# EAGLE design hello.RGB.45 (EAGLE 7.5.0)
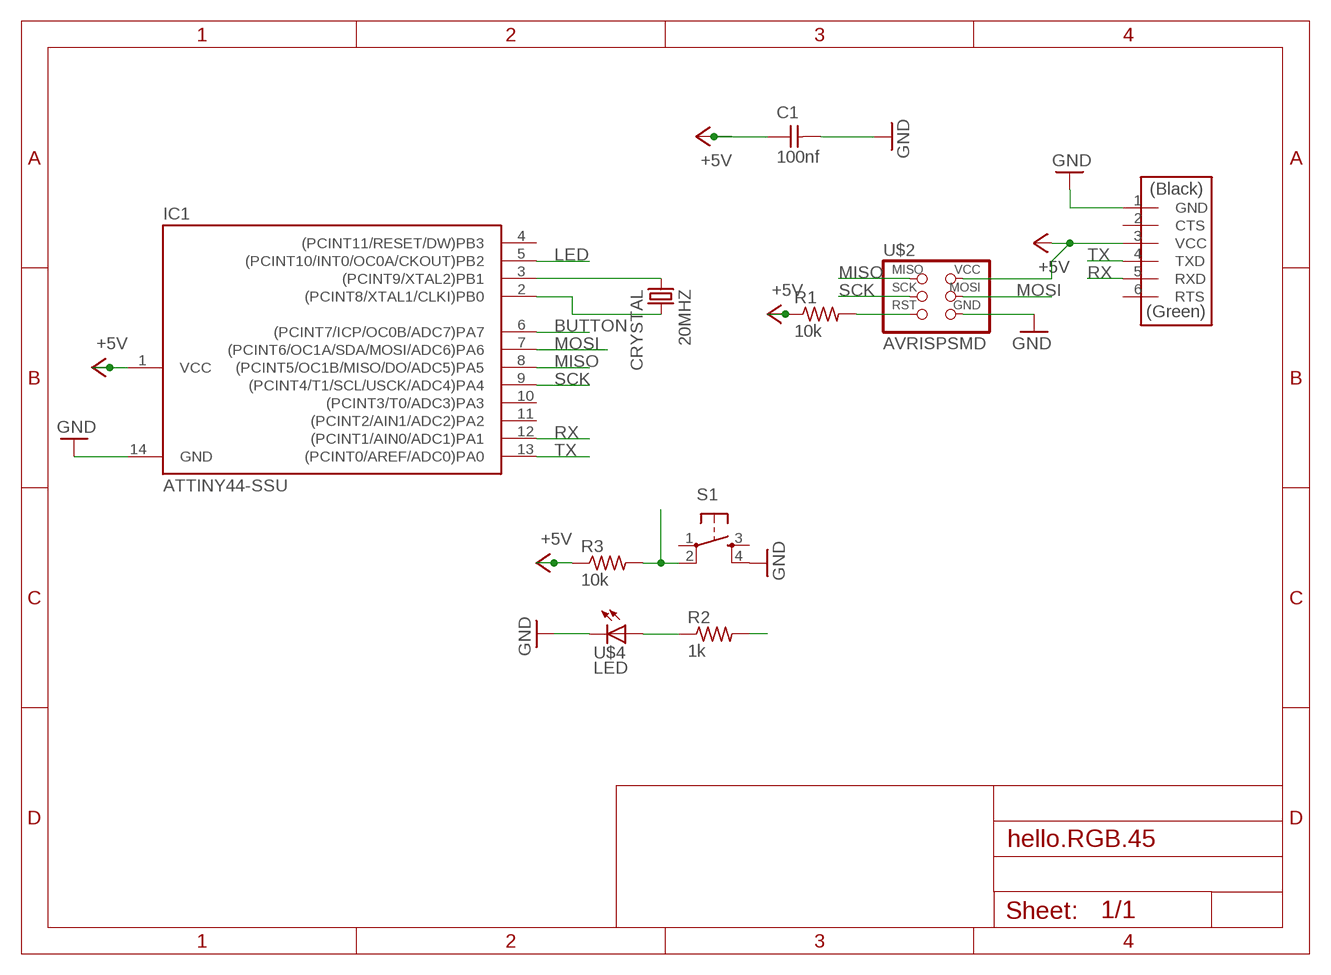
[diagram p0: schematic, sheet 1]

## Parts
20MHZ  CRYSTAL  [2-SMD-5X3MM]
C1  100nf  CAP-UNPOLARIZEDFAB  [C1206FAB]
IC1  ATTINY44-SSU  [SOIC14]
R1  10k  RES-US1206  [R1206]
R2  1k  RES-US1206  [R1206]
R3  10k  RES-US1206  [R1206]
S1  6MM_SWITCH6MM_SWITCH  [6MM_SWITCH]
U$1  FTDI-SMD-HEADER  [1X06SMD]
U$2  AVRISPSMD  [2X03SMD]
U$4  LED  [LED1206]

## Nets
+5V: C1.1 IC1.1(VCC) R1.1 R3.1 U$1.3(VCC) U$2.2(VCC)
BUTTON: IC1.6((PCINT7/ICP/OC0B/ADC7)PA7) R3.2 S1.2(P1)
GND: C1.2 IC1.14(GND) S1.4(S1) U$1.1(GND) U$2.6(GND) U$4.2(C)
LED: IC1.5((PCINT10/INT0/OC0A/CKOUT)PB2) R2.2
MISO: IC1.8((PCINT5/OC1B/MISO/DO/ADC5)PA5) U$2.1(MISO)
MOSI: IC1.7((PCINT6/OC1A/SDA/MOSI/ADC6)PA6) U$2.4(MOSI)
N$1: 20MHZ.P$2 IC1.2((PCINT8/XTAL1/CLKI)PB0)
N$2: 20MHZ.P$1 IC1.3((PCINT9/XTAL2)PB1)
N$11: R1.2 U$2.5(RST)
N$14: R2.1 U$4.1(A)
RX: IC1.12((PCINT1/AIN0/ADC1)PA1) U$1.5(RXD)
SCK: IC1.9((PCINT4/T1/SCL/USCK/ADC4)PA4) U$2.3(SCK)
TX: IC1.13((PCINT0/AREF/ADC0)PA0) U$1.4(TXD)
Unconnected: IC1.4((PCINT11/RESET/DW)PB3) IC1.10((PCINT3/T0/ADC3)PA3) IC1.11((PCINT2/AIN1/ADC2)PA2) S1.1(P) S1.3(S) U$1.2(CTS) U$1.6(RTS)

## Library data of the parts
20MHZ = fab:CRYSTAL
C1 = fab:CAP-UNPOLARIZED
IC1 = fab:ATTINY44
R1-R3 = fab:RES-US: Resistor (US Symbol)
S1 = fab:6MM_SWITCH: OMRON SWITCH
U$1 = fab:FTDI-SMD-HEADER
U$2 = fab:AVRISP
U$4 = fab:LED: LED

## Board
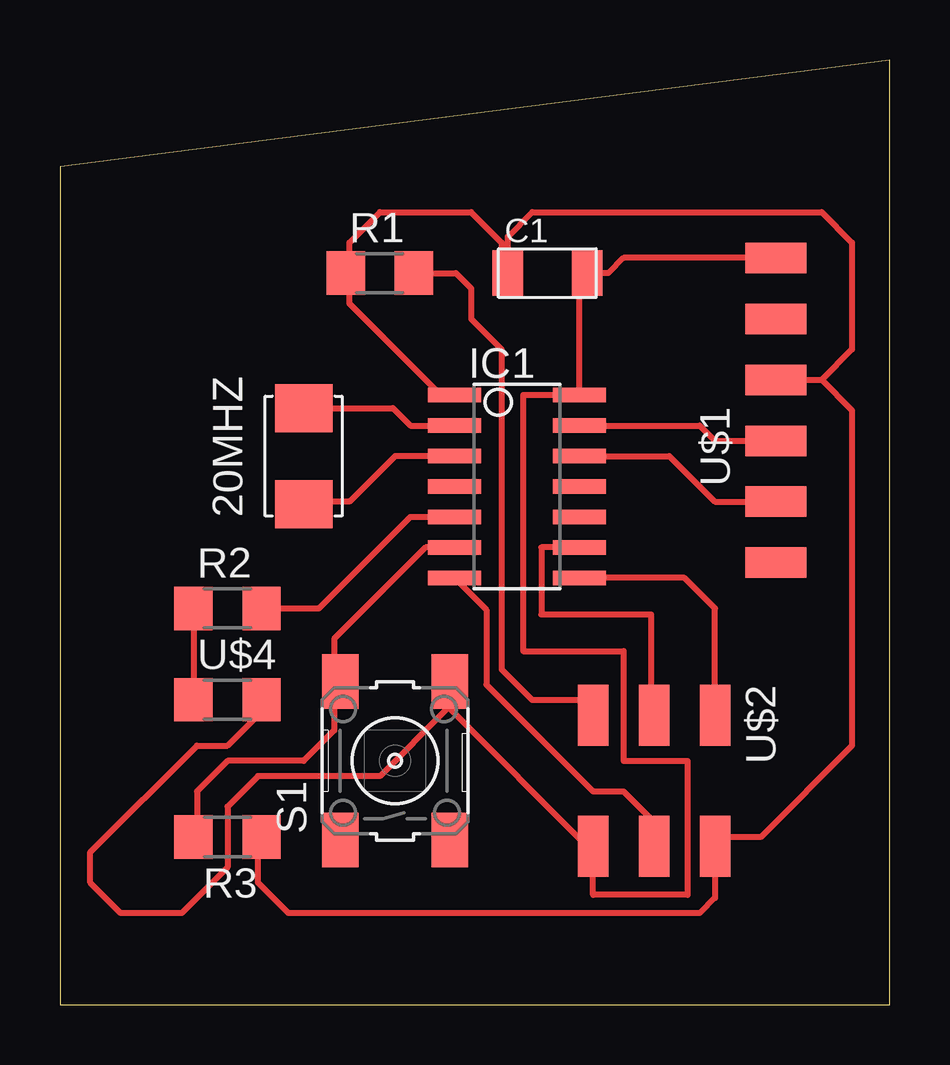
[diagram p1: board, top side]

Size 34.59 x 39.36 mm. Coordinates in mm from the lower left corner, seen from the top.
Outline: 0,0 34.59,0 34.59,39.36 0,34.92 0,0
Copper layers (1*16): Top 0.035mm / dielectric 1.5mm / Bottom 0.035mm
Design rules "default": minimum track width 10mil, minimum drill 24mil, track to track 8mil, track to pad 8mil, pad to pad 8mil, via to via 8mil, smd to smd 8mil, copper to edge 40mil, drill to drill 8mil, minimum pad ring 10mil, minimum via ring 8mil, stop-mask expansion 4mil, vias tented up to drill 0mil, thermal gap 10mil

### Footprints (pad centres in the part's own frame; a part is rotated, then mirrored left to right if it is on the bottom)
2-SMD-5X3MM = smd 2 x 2.4: P$1 -2,0; P$2 2,0
C1206FAB = smd 1.27 x 1.905: 1 -1.651,0; 2 1.651,0
SOIC14 = smd 0.61 x 2.21: 1 -3.81,-2.603; 2 -2.54,-2.603; 3 -1.27,-2.603; 4 0,-2.603; 5 1.27,-2.603; 6 2.54,-2.603; 7 3.81,-2.603; 8 3.81,2.603; 9 2.54,2.603; 10 1.27,2.603; 11 0,2.603; 12 -1.27,2.603; 13 -2.54,2.603; 14 -3.81,2.603
R1206 = smd 1.6 x 1.803: 1 -1.422,0; 2 1.422,0
6MM_SWITCH = smd 2.286 x 1.524: 1 -3.302,2.286; 2 3.302,2.286; 3 -3.302,-2.286; 4 3.302,-2.286
1X06SMD = smd 2.54 x 1.27: 1 0,6.35; 2 0,3.81; 3 0,1.27; 4 0,-1.27; 5 0,-3.81; 6 0,-6.35
2X03SMD = smd 2.54 x 1.27: 1 -2.54,2.54; 2 2.92,2.54; 3 -2.54,0; 4 2.92,0; 5 -2.54,-2.54; 6 2.92,-2.54
LED1206 = smd 1.6 x 1.803: 1 -1.422,0; 2 1.422,0

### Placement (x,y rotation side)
20MHZ  10.16,22.86 90 top
C1  20.32,30.48 0 top
IC1  19.05,21.59 270 top
R1  13.34,30.48 0 top
R2  6.99,16.51 0 top
R3  6.99,6.98 180 top
S1  13.97,10.16 90 top
U$1  29.84,24.77 0 top
U$2  24.77,9.52 270 top
U$4  6.99,12.7 0 top

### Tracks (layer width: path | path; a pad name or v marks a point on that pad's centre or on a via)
+5V
  Top 0.254: IC1.1 15.88,25.4 12.06,29.21 12.06,30.33 | 12.06,30.33 12.06,31.75 13.34,33.02 17.14,33.02 18.41,31.75 18.41,30.73 C1.1 18.67,32 19.68,33.02 31.75,33.02 33.02,31.75 33.02,27.3 31.75,26.03 | U$1.3 31.75,26.03 | 31.75,26.03 33.02,24.77 33.02,10.8 29.21,6.98 27.68,6.98 U$2.2 27.3,4.45 26.67,3.81 9.53,3.81 8.26,5.08 8.26,6.83 R3.1 | 12.06,30.33 R1.1
BUTTON
  Top 0.254: R3.2 5.71,7.14 5.71,8.89 6.99,10.16 10.16,10.16 11.43,11.43 11.43,13.72 | IC1.6 15.24,19.05 11.43,15.24 11.43,13.72 | 11.43,13.72 S1.2
GND
  Top 0.254: U$1.1 23.5,31.11 22.86,30.48 C1.2 21.65,30.16 IC1.14 19.3,25.4 19.3,14.73 23.5,14.73 23.5,10.16 26.16,10.16 26.16,4.57 22.23,4.57 U$2.6 | S1.4 16.26,12.32 | 16.26,12.32 21.97,6.6 U$2.6 | 16.26,12.32 16.13,12.32 13.34,9.52 8.26,9.52 6.99,8.26 6.99,5.71 5.08,3.81 2.54,3.81 1.27,5.08 1.27,6.35 5.71,10.8 6.99,10.8 8.26,12.06 8.26,12.55 U$4.2 | U$2.6
LED
  Top 0.254: R2.2 10.79,16.51 14.61,20.32 IC1.5
MISO
  Top 0.254: U$2.1 27.3,16.51 26.04,17.78 IC1.8
MOSI
  Top 0.254: IC1.7 17.78,16.45 17.78,13.34 22.23,8.89 23.5,8.89 24.77,7.62 U$2.4
N$1
  Top 0.254: 20MHZ.P$2 13.88,24.86 14.61,24.13 IC1.2
N$2
  Top 0.254: IC1.3 13.97,22.86 12.06,20.95 10.26,20.95 20MHZ.P$1
N$11
  Top 0.254: R1.2 16.51,30.48 17.14,29.84 17.14,28.58 18.41,27.3 18.41,13.97 19.68,12.7 21.59,12.7 U$2.5
N$14
  Top 0.254: R2.1 U$4.1
RX
  Top 0.254: IC1.12 25.4,22.86 27.3,20.95 U$1.5
SCK
  Top 0.254: IC1.9 20.07,19.05 20.07,16.26 24.64,16.26 24.64,12.95 24.77,12.95 U$2.3
TX
  Top 0.254: IC1.13 26.67,24.13 27.3,23.5 U$1.4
